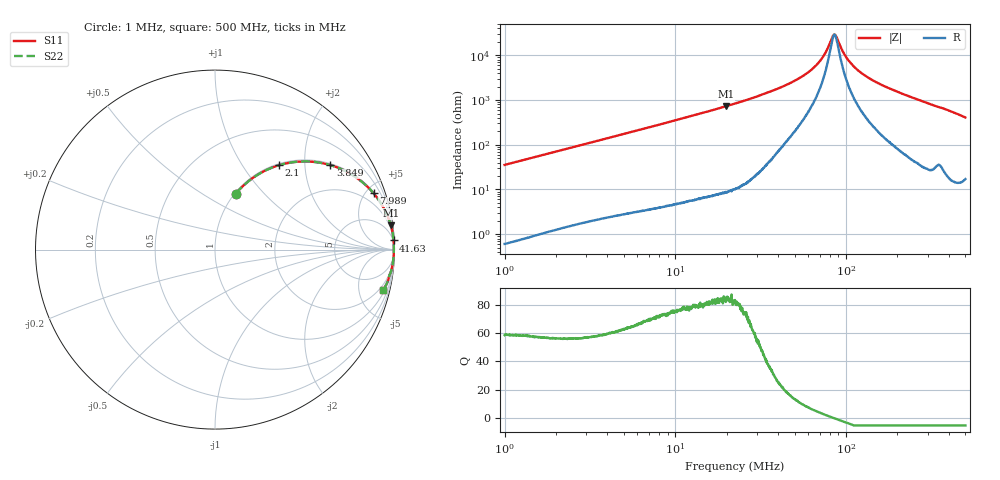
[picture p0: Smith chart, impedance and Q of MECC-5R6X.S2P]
!s-Parameter Generated by FASTRON Sdn. Bhd.
!FASTRON P/N : MECC-5R6X
!Keysight Technologies,E4991B,MY54100416,A.01.15
!Date: Thu Apr 02 10:32:07 2026
!Version  : Rev00 Thu Apr 02 10:32:07 2026
!Data & Calibration Information:
!PortZ  Port1:50+j0  Port2:50+j0
!When reading, reference impedance value at option line is always used.
!Remarks : This data is being provided solely for informational purposes.
!Freq	S11	S21	S12	S22
# Hz S dB R 50
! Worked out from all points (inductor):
!   1601 points, 1 MHz to 500 MHz, reference 50 ohm
!   read as one part in series: L = 5.63 uH near 1.032 MHz
!   highest Q = 84 at 19.82 MHz (marker M1), where L = 5.83 uH
!   self-resonance near 85.4 MHz
!   S11 on the Smith chart (normalised r, x): 1 MHz: 1.01, +0.71; 2.1 MHz: 1.03, +1.48; 3.849 MHz: 1.05, +2.69; 7.989 MHz: 1.08, +5.59; 41.63 MHz: 3, +39; 500 MHz: 1.34, -8.14
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1000000  -9.57 69.6  -0.56 -19.4  -0.56 -19.4  -9.57 69.6
2099856  -4.59 52.9  -1.97 -36.1  -1.97 -36.1  -4.59 52.9
2820919  -3.13 44.8  -3.04 -44.2  -3.04 -44.2  -3.13 44.8
3848922  -1.98 36.2  -4.56 -52.8  -4.56 -52.8  -1.98 36.2
7957584  -0.57 19.7  -9.46 -69.5  -9.46 -69.5  -0.57 19.7
7988553  -0.56 19.6  -9.49 -69.6  -9.49 -69.6  -0.56 19.6
1.982405e7  -0.10 7.8  -17.32 -81.5  -17.32 -81.5  -0.10 7.8
2.236068e7  -0.07 6.8  -18.49 -82.5  -18.49 -82.5  -0.07 6.8
4.162766e7  -0.03 2.9  -25.76 -84.5  -25.76 -84.5  -0.03 2.9
5.275702e7  -0.03 1.9  -29.63 -83.1  -29.63 -83.1  -0.03 1.9
6.307767e7  -0.03 1.2  -33.76 -79.9  -33.76 -79.9  -0.03 1.2
7.254416e7  -0.03 0.6  -38.88 -72.5  -38.88 -72.5  -0.03 0.6
7.689627e7  -0.03 0.4  -42.13 -63.8  -42.13 -63.8  -0.03 0.4
8.310792e7  -0.03 0.1  -48.13 -28.6  -48.13 -28.6  -0.03 0.1
8.573088e7  -0.03 -0.0  -49.30 1.8  -49.30 1.8  -0.03 -0.0
8.809378e7  -0.03 -0.1  -48.06 28.6  -48.06 28.6  -0.03 -0.1
9.9366e7  -0.03 -0.6  -39.60 69.9  -39.60 69.9  -0.03 -0.6
1.120806e8  -0.03 -1.0  -34.74 78.0  -34.74 78.0  -0.03 -1.0
1.361047e8  -0.03 -1.8  -29.85 82.1  -29.85 82.1  -0.03 -1.8
1.77937e8  -0.04 -3.1  -25.35 83.3  -25.35 83.3  -0.04 -3.1
3.608063e8  -0.15 -8.4  -16.71 78.9  -16.71 78.9  -0.15 -8.4
5e8  -0.34 -13.6  -12.54 73.9  -12.54 73.9  -0.34 -13.6
